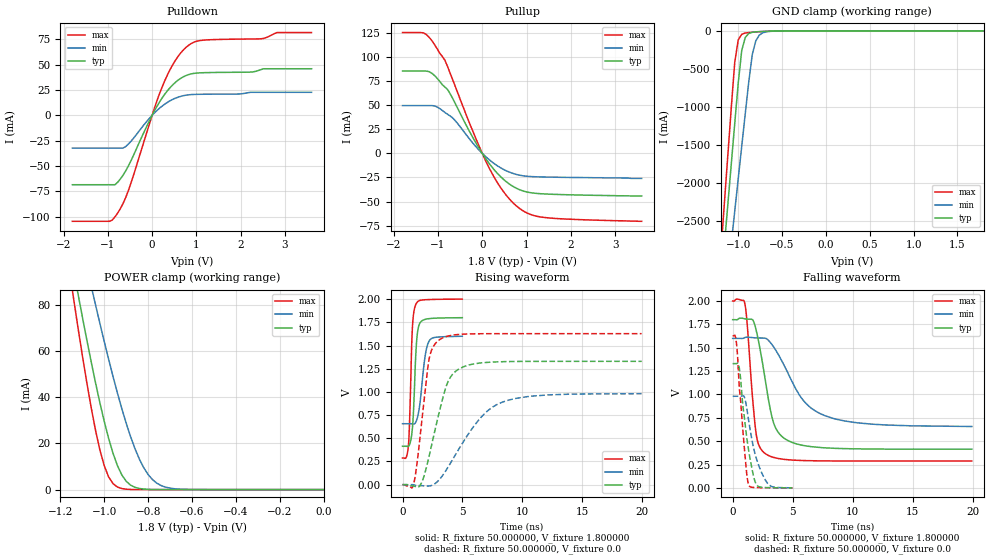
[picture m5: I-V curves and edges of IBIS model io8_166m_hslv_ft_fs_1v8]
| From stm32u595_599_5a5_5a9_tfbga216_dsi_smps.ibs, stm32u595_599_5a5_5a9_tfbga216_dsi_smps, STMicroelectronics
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|   Model io8_166m_hslv_ft_fs_1v8
[Model]  io8_166m_hslv_ft_fs_1v8
Model_type I/O
Polarity   Non-Inverting
Enable   Active-Low
Vinl =   0.540000V
Vinh =   1.260000V
Vmeas =  0.900000V
Cref =   50.000000pF
Rref =   100.000000M
Vref =   0.0V
C_comp   3.358400pF   3.352800pF   3.400400pF
[Temperature Range]   25.000000   0.140000k   -40.000000
[Pullup Reference]   1.800000V   1.600000V   2.000000V
[Pulldown Reference]   0.0V   0.0V   0.0V
[POWER Clamp Reference]   1.800000V   1.600000V   2.000000V
[GND Clamp Reference]   0.0V   0.0V   0.0V
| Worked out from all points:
|   slope of the pulldown table from 0 to 0.27 V, typ, clamps not added: 13.6 ohm
|   slope of the pullup table from 0 to 0.27 V, typ, clamps not added: 15.9 ohm
|   GND clamp passes 1 mA (typ) near -0.51 V on its own axis
|   POWER clamp passes 1 mA (typ) near -0.86 V on its own axis
|   rising waveform, R_fixture 50.000000, V_fixture 1.800000: 20-80 % time 290ps typ, 498ps min, 237ps max; typ from 0.414 V to 1.8 V
|   rising waveform, R_fixture 50.000000, V_fixture 0.0: 20-80 % time 1.51ns typ, 3.17ns min, 854ps max; typ from 0 V to 1.33 V
|   falling waveform, R_fixture 50.000000, V_fixture 1.800000: 20-80 % time 1.2ns typ, 2.76ns min, 638ps max; typ from 1.8 V to 0.414 V
|   falling waveform, R_fixture 50.000000, V_fixture 0.0: 20-80 % time 788ps typ, 1.05ns min, 590ps max; typ from 1.33 V to 0 V
[Pulldown]
|Voltage   I(typ)   I(min)   I(max)
-1.8V     -68.38mA   -32.32mA   -104.4mA
-960mV    -68.38mA   -32.32mA   -104.4mA
-780mV    -66.08mA   -32.32mA   -96.42mA
-540mV    -50.22mA   -28.51mA   -74.66mA
0V        0A         -400fA     0A
240mV     18.04mA    9.6mA      29.42mA
480mV     30.68mA    16.02mA    50.95mA
780mV     39.48mA    19.99mA    67.57mA
1.14V     41.99mA    20.78mA    74.01mA
2.46V     45.09mA    22.69mA    75.45mA
2.82V     45.91mA    22.69mA    81.58mA
3.6V      45.91mA    22.69mA    81.58mA
[Pullup]
|Voltage   I(typ)   I(min)   I(max)
-1.8V     85.37mA    49.56mA    125.3mA
-1.32V    85.37mA    49.56mA    124.9mA
-1.08V    80.85mA    49.28mA    113.1mA
-840mV    68.71mA    42.35mA    96.4mA
-660mV    56.31mA    36.43mA    75.51mA
-180mV    13.77mA    8.913mA    19.32mA
180mV     -11.9mA    -7.442mA   -17.26mA
480mV     -26.98mA   -16.65mA   -39.76mA
840mV     -37.65mA   -22.63mA   -57.07mA
1.08V     -40.74mA   -24.01mA   -63.22mA
1.44V     -42.19mA   -24.58mA   -66.73mA
3.6V      -44.2mA    -26mA      -70.5mA
[GND_clamp]
|Voltage   I(typ)   I(min)   I(max)
-1.8V     -9.908A    -9.683A    -9.994A
-1.2V     -3.383A    -4.084A    -2.934A
-1.16V    -2.841A    -3.655A    -2.294A
-1.12V    -2.299A    -3.226A    -1.656A
-1.04V    -1.218A    -2.369A    -414.2mA
-1V       -684.7mA   -1.941A    -119.2mA
-960mV    -257.2mA   -1.514A    -45.66mA
-920mV    -87.03mA   -1.089A    -28.93mA
-840mV    -19.35mA   -312.8mA   -18.97mA
-800mV    -13.55mA   -132.4mA   -15.49mA
-720mV    -8.042mA   -25.67mA   -9.491mA
1.8V      0A         13.64nA    0A
[POWER_clamp]
|Voltage   I(typ)   I(min)   I(max)
-1.8V     470.8mA    433.7mA    554.6mA
-1.14V    95.25mA    122.7mA    82.82mA
-1.12V    84.97mA    114mA      70.27mA
-1.06V    55.51mA    88.42mA    35.67mA
-1.04V    46.34mA    80.15mA    25.76mA
-1V       29.51mA    64.13mA    10.3mA
-940mV    10.39mA    41.86mA    1.109mA
-900mV    3.624mA    28.77mA    182.8uA
-840mV    490.7uA    13.24mA    11.35uA
-800mV    116.8uA    6.532mA    1.77uA
-740mV    13.2uA     1.724mA    109.3nA
0V        0A         18.75nA    0A
[Ramp]
| variable   typ   min   max
dV/dt_r  0.79770/1.50752n   0.58789/3.16284n   0.97662/0.85234n
dV/dt_f  0.83164/1.19722n   0.56479/2.75302n   1.02770/0.63637n
R_load = 50.000000
[Rising Waveform]
R_fixture= 50.000000
V_fixture= 1.800000
V_fixture_min= 1.600000
V_fixture_max= 2.000000
|time   V(typ)   V(min)   V(max)
0s        413.9mV    656.9mV    287.2mV
500.5ps   412.8mV    657mV      437.3mV
590.6ps   433.1mV    657mV      694.3mV
810.8ps   591.6mV    655.8mV    1.659V
1.071ns   1.306V     665.6mV    1.931V
1.211ns   1.599V     710.3mV    1.965V
1.371ns   1.718V     804.8mV    1.982V
1.872ns   1.781V     1.375V     1.993V
2.192ns   1.789V     1.544V     1.995V
4.985ns   1.8V       1.6V       2V
[Rising Waveform]
R_fixture= 50.000000
V_fixture= 0.0
V_fixture_min= 0.0
V_fixture_max= 0.0
|time   V(typ)   V(min)   V(max)
0s        -26.75uV   -4.209uV   -6.921uV
920.9ps   -14.89mV   -1.619mV   3.034mV
1.562ns   13.8mV     -10.95mV   633.6mV
2.202ns   299.1mV    -14.1mV    1.344V
3.163ns   835.3mV    68.93mV    1.57V
3.804ns   1.114V     191.3mV    1.603V
4.484ns   1.228V     338.4mV    1.617V
6.607ns   1.313V     734.6mV    1.627V
8.368ns   1.326V     891.8mV    1.628V
19.94ns   1.33V      980.4mV    1.628V
[Falling Waveform]
R_fixture= 50.000000
V_fixture= 1.800000
V_fixture_min= 1.600000
V_fixture_max= 2.000000
|time   V(typ)   V(min)   V(max)
0s        1.8V       1.6V       2V
1.001ns   1.81V      1.608V     1.98V
1.201ns   1.807V     1.613V     1.769V
1.962ns   1.687V     1.605V     575.5mV
2.763ns   1.12V      1.6V       363mV
3.363ns   717mV      1.518V     327.8mV
4.004ns   562.8mV    1.382V     310.4mV
5.846ns   454.9mV    943.5mV    292.3mV
7.688ns   428.5mV    772.7mV    288.6mV
19.94ns   413.9mV    656.9mV    287.2mV
[Falling Waveform]
R_fixture= 50.000000
V_fixture= 0.0
V_fixture_min= 0.0
V_fixture_max= 0.0
|time   V(typ)   V(min)   V(max)
0s        1.33V      980.4mV    1.628V
290.3ps   1.33V      980.4mV    1.575V
400.4ps   1.335V     980.5mV    1.428V
530.5ps   1.299V     980.5mV    1.129V
981ps     750.7mV    970.2mV    420.4mV
1.191ns   524.5mV    839.9mV    131.1mV
1.341ns   395.1mV    715.7mV    32.05mV
1.952ns   42.05mV    325.4mV    2.9mV
2.773ns   3.099mV    73.68mV    1.115mV
4.985ns   -26.75uV   -4.209uV   -6.921uV
